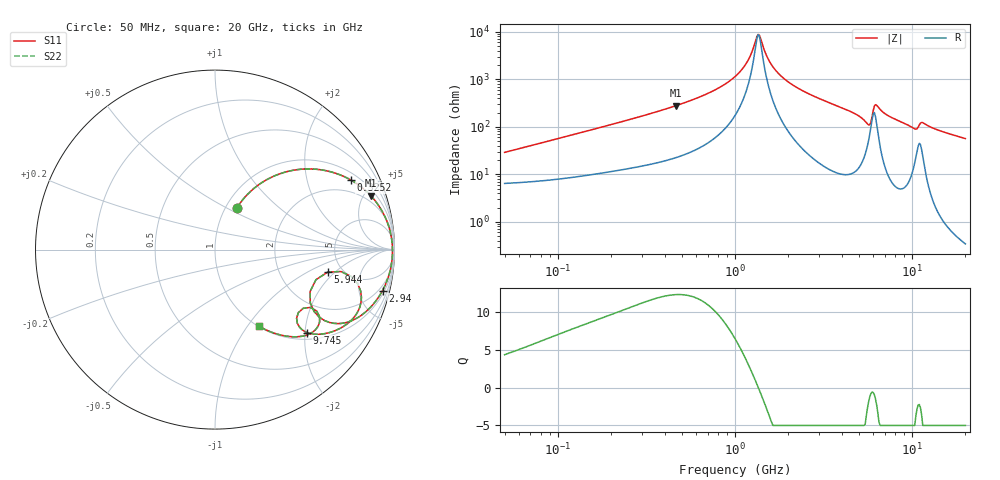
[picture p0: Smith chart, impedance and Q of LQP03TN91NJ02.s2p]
!Murata Part Number: LQP03TN91NJ02
!These Parameters are Measured in Series Mode Connection
!  o--[Z]--o
!Port1  Port2
!  o-------o
!Freq. Start=50[MHz] Stop=20[GHz], 401[Steps]
# Hz S RI R 50
!Freq.(Hz) S11(Real) S11(Imag) S21(Real) S21(Imag) S12(Real) S12(Imag) S22(Real) S22(Imag)
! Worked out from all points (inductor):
!   401 points, 50 MHz to 20 GHz, reference 50 ohm
!   read as one part in series: L = 89.4 nH near 51.52 MHz
!   highest Q = 12.4 at 465.8 MHz (marker M1), where L = 95.4 nH
!   self-resonance near 1.349 GHz
!   S11 on the Smith chart (normalised r, x): 50 MHz: 1.13, +0.57; 325.2 MHz: 1.32, +3.68; 2.94 GHz: 1.36, -8.08; 5.944 GHz: 3.82, -1.62; 9.745 GHz: 1.16, -2.05; 20 GHz: 1.01, -1.13
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5e7  0.1223 0.2331  0.8777 -0.2331  0.8777 -0.2331  0.1223 0.2331
1.364002e8  0.3826 0.4294  0.6174 -0.4294  0.6174 -0.4294  0.3826 0.4294
3.251725e8  0.7552 0.3889  0.2448 -0.3889  0.2448 -0.3889  0.7552 0.3889
3.721004e8  0.8025 0.3586  0.1975 -0.3586  0.1975 -0.3586  0.8025 0.3586
4.658406e8  0.8682 0.3003  0.1318 -0.3003  0.1318 -0.3003  0.8682 0.3003
7.411344e8  0.9537 0.1681  0.0463 -0.1681  0.0463 -0.1681  0.9537 0.1681
1e9  0.9797 0.0839  0.0203 -0.0839  0.0203 -0.0839  0.9797 0.0839
1.161586e9  0.9862 0.0425  0.0138 -0.0425  0.0138 -0.0425  0.9862 0.0425
1.369645e9  0.9889 -0.00279  0.0111 0.00279  0.0111 0.00279  0.9889 -0.00279
1.544007e9  0.988 -0.036  0.012 0.036  0.012 0.036  0.988 -0.036
1.740566e9  0.9847 -0.0696  0.0153 0.0696  0.0153 0.0696  0.9847 -0.0696
2.728004e9  0.9454 -0.204  0.0546 0.204  0.0546 0.204  0.9454 -0.204
2.940159e9  0.9334 -0.2282  0.0666 0.2282  0.0666 0.2282  0.9334 -0.2282
5.194772e9  0.6823 -0.4122  0.3177 0.4122  0.3177 0.4122  0.6823 -0.4122
5.683258e9  0.531 -0.2974  0.469 0.2974  0.469 0.2974  0.531 -0.2974
5.944466e9  0.6274 -0.1254  0.3726 0.1254  0.3726 0.1254  0.6274 -0.1254
6.406762e9  0.8159 -0.2659  0.1841 0.2659  0.1841 0.2659  0.8159 -0.2659
7.442007e9  0.7243 -0.4226  0.2757 0.4226  0.2757 0.4226  0.7243 -0.4226
9.745021e9  0.5135 -0.4624  0.4865 0.4624  0.4865 0.4624  0.5135 -0.4624
1.082228e10  0.4921 -0.3266  0.5079 0.3266  0.5079 0.3266  0.4921 -0.3266
1.166392e10  0.5741 -0.4274  0.4259 0.4274  0.4259 0.4274  0.5741 -0.4274
2e10  0.2435 -0.4262  0.7565 0.4262  0.7565 0.4262  0.2435 -0.4262
